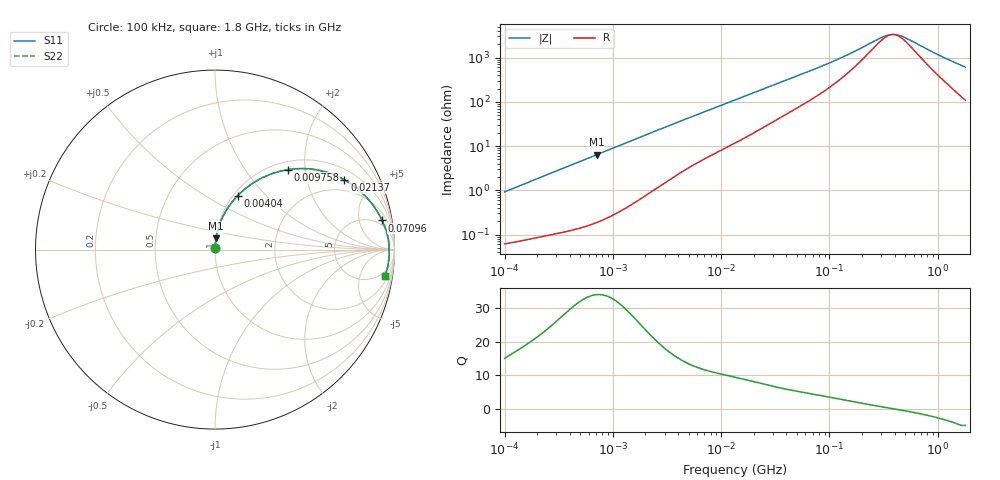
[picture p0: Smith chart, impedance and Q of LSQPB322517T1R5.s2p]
! LSQPB322517T1R5  S-PARAMETER MODEL  ( General Type )
! Model Generated by TAIYO YUDEN Corporation (http://www.ty-top.com)
! Version 2.0
! TAIYO YUDEN Control No. 100810NG22EB-FKC
! Copyright(c) 2009 TAIYO YUDEN CO.,LTD. All Rights Reserved.
! Product Description (link to TY-COMPAS)
! https://ds.yuden.co.jp/TYCOMPAS/or/detail?pn=LSQPB322517T1R5M&u=M
! Products Name : Inductors
! Characteristics :
!  Inductance : 1.5 uH , SRF(min) : 170 MHz , DC Resistance(max) : 0.054 Ohm
!  Rated Current : Saturation :2200 mA , Temp Rise : 1750 mA (40 degC)
!  Case Size : 3.2 x 2.5 / 0.126 x 0.098 [mm/inch] , Thickness : 1.7 / 0.068 [mm/inch]
!  (Conditions: Temperature = 25 degC , DC Bias Current/Voltage = 0A / 0V)
! External Node Assignments :
!  1  o---GGG---o  2
! GND o---------o GND
! Frequency Range : 0.1MHz  -  1800MHz  [ 402 STEP ]
# MHz S RI R 50
! Freq[MHz].  S11 Real  S11 Imag  S21 Real  S21 Imag  S12 Real  S12 Imag  S22 Real  S22 Imag
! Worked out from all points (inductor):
!   401 points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, 100 kHz to 1.8 GHz, reference 50 ohm
!   read as one part in series: L = 1.46 uH near 105 kHz
!   highest Q = 34 at 709.7 kHz (marker M1), where L = 1.43 uH
!   self-resonance near 384.2 MHz
!   S11 on the Smith chart (normalised r, x): 100 kHz: 1.00, +0.02; 4.04 MHz: 1.05, +0.70; 9.758 MHz: 1.16, +1.62; 21.37 MHz: 1.43, +3.40; 70.96 MHz: 3, +10; 1.8 GHz: 3, -12
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0.1  0.000698 0.0092  0.9993 -0.0092  0.9993 -0.0092  0.000698 0.0092
0.516129  0.00357 0.0462  0.9964 -0.0462  0.9964 -0.0462  0.00357 0.0462
0.709667  0.00588 0.0632  0.9941 -0.0632  0.9941 -0.0632  0.00588 0.0632
1.409041  0.0197 0.1228  0.9803 -0.1228  0.9803 -0.1228  0.0197 0.1228
2.66389  0.0626 0.218  0.9374 -0.218  0.9374 -0.218  0.0626 0.218
4.039851  0.1262 0.3004  0.8738 -0.3004  0.8738 -0.3004  0.1262 0.3004
6.126528  0.2336 0.3841  0.7664 -0.3841  0.7664 -0.3841  0.2336 0.3841
9.75753  0.4074 0.4456  0.5926 -0.4456  0.5926 -0.4456  0.4074 0.4456
13.41641  0.5436 0.4477  0.4564 -0.4477  0.4564 -0.4477  0.5436 0.4477
21.36789  0.7214 0.3889  0.2786 -0.3889  0.2786 -0.3889  0.7214 0.3889
27.97575  0.7979 0.3355  0.2021 -0.3355  0.2021 -0.3355  0.7979 0.3355
36.62703  0.8541 0.28  0.1459 -0.28  0.1459 -0.28  0.8541 0.28
69.24595  0.9295 0.1663  0.0705 -0.1663  0.0705 -0.1663  0.9295 0.1663
70.9631  0.9312 0.1626  0.0688 -0.1626  0.0688 -0.1626  0.9312 0.1626
130.9143  0.9594 0.0858  0.0406 -0.0858  0.0406 -0.0858  0.9594 0.0858
180.0045  0.9657 0.056  0.0343 -0.056  0.0343 -0.056  0.9657 0.056
293.7968  0.9701 0.0184  0.0299 -0.0184  0.0299 -0.0184  0.9701 0.0184
357.3983  0.9707 0.00493  0.0293 -0.00493  0.0293 -0.00493  0.9707 0.00493
413.9822  0.9709 -0.00509  0.0291 0.00509  0.0291 0.00509  0.9709 -0.00509
479.5244  0.9708 -0.0152  0.0292 0.0152  0.0292 0.0152  0.9708 -0.0152
1024.694  0.9651 -0.0778  0.0349 0.0778  0.0349 0.0778  0.9651 -0.0778
1800  0.9479 -0.1491  0.0521 0.1491  0.0521 0.1491  0.9479 -0.1491
